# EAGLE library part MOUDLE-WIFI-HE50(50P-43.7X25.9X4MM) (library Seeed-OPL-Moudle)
317060007
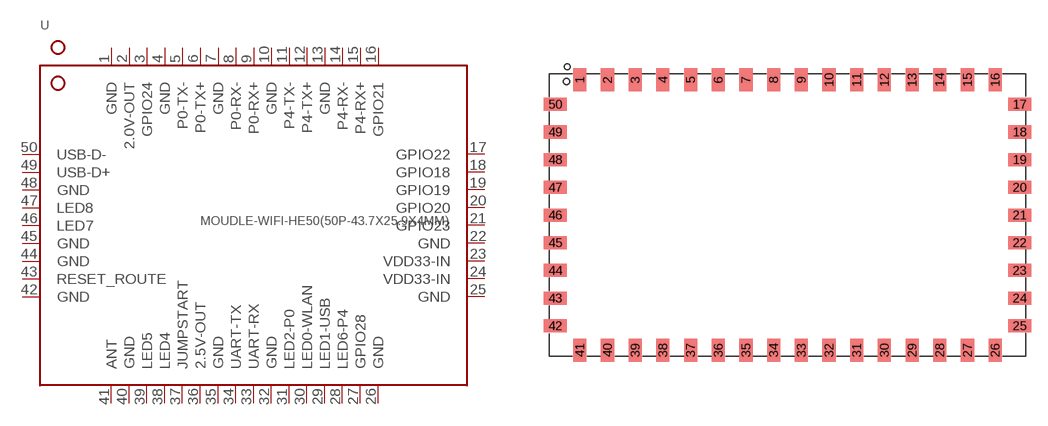
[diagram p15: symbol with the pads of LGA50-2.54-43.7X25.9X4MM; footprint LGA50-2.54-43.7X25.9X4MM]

Designator prefix U

## MOUDLE-WIFI-HE50(50P-43.7X25.9X4MM) (MPN: HE50; VALUE: HE50)  [LGA50-2.54-43.7X25.9X4MM]
1  GND  sup
2  2.0V-OUT
3  GPIO24
4  GND  sup
5  P0-TX-
6  P0-TX+
7  GND  sup
8  P0-RX-
9  P0-RX+
10  GND  sup
11  P4-TX-
12  P4-TX+
13  GND
14  P4-RX-
15  P4-RX+
16  GPIO21
17  GPIO22
18  GPIO18
19  GPIO19
20  GPIO20
21  GPIO23
22  GND  sup
23  VDD33-IN  pwr
24  VDD33-IN  pwr
25  GND  sup
26  GND  sup
27  GPIO28
28  LED6-P4
29  LED1-USB
30  LED0-WLAN
31  LED2-P0
32  GND  sup
33  UART-RX
34  UART-TX
35  GND  sup
36  2.5V-OUT  pwr
37  JUMPSTART
38  LED4
39  LED5
40  GND  sup
41  ANT
42  GND  sup
43  RESET_ROUTE
44  GND  sup
45  GND  sup
46  LED7
47  LED8
48  GND  sup
49  USB-D+
50  USB-D-

## Footprint LGA50-2.54-43.7X25.9X4MM (pad centres in mm)
smd 1.2 x 2.1: 1 -19.05,12.4; 2 -16.51,12.4; 3 -13.97,12.4; 4 -11.43,12.4; 5 -8.89,12.4; 6 -6.35,12.4; 7 -3.81,12.4; 8 -1.27,12.4; 9 1.27,12.4; 10 3.81,12.4; 11 6.35,12.4; 12 8.89,12.4; 13 11.43,12.4; 14 13.97,12.4; 15 16.51,12.4; 16 19.05,12.4; 26 19.05,-12.4; 27 16.51,-12.4; 28 13.97,-12.4; 29 11.43,-12.4; 30 8.89,-12.4; 31 6.35,-12.4; 32 3.81,-12.4; 33 1.27,-12.4; 34 -1.27,-12.4; 35 -3.81,-12.4; 36 -6.35,-12.4; 37 -8.89,-12.4; 38 -11.43,-12.4; 39 -13.97,-12.4; 40 -16.51,-12.4; 41 -19.05,-12.4
smd 2.1 x 1.2: 17 21.3,10.16; 18 21.3,7.62; 19 21.3,5.08; 20 21.3,2.54; 21 21.3,0; 22 21.3,-2.54; 23 21.3,-5.08; 24 21.3,-7.62; 25 21.3,-10.16; 42 -21.3,-10.16; 43 -21.3,-7.62; 44 -21.3,-5.08; 45 -21.3,-2.54; 46 -21.3,0; 47 -21.3,2.54; 48 -21.3,5.08; 49 -21.3,7.62; 50 -21.3,10.16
